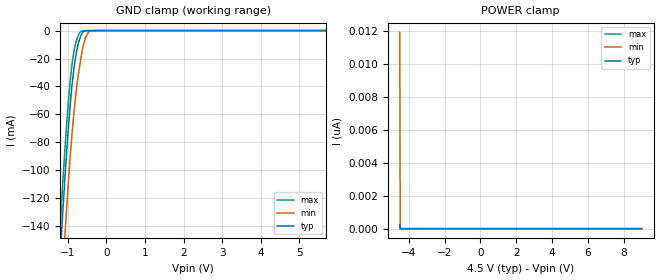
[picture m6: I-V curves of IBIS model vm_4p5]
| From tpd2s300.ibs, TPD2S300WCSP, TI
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|   VM_4p5 Model
[Model]   vm_4p5
Model_type   Input
Vinl = 1.35
Vinh = 3.15
|   typ   min   max
C_comp   15.123pF   11.1308pF   19.254pF
[Model spec]
|subparameter
Vinl   1.35   1.3497   1.3503
Vinh   3.15   3.1493   3.1507
| Where nom  PVT is Nominal Process, 4.5V, 27C
|   Fast PVT is Strong Process,  4.501V, -40C
|   Slow PVT is Weak Process,   4.499V, 125C
[Voltage Range]   4.5   4.499   4.501
[Temperature Range]   27   125   -40
[Power Clamp Reference]   4.5   4.499   4.501
[GND Clamp Reference]   0   0   0
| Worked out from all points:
|   GND clamp passes 1 mA (typ) near -0.60 V on its own axis
[GND Clamp]
|   Voltage   I(typ)   I(min)   I(max)
-4.5V     -1.887A    -2.023A    -1.826A
-1.26V    -189.6mA   -234.2mA   -167.6mA
-1.125V   -126.8mA   -169.1mA   -105.7mA
-1.058V   -97.56mA   -138.5mA   -77.21mA
-949.5mV  -56.44mA   -94.23mA   -38.92mA
-868.5mV  -33.11mA   -66.44mA   -19.36mA
-774mV    -15.04mA   -41.26mA   -6.877mA
-652.5mV  -3.023mA   -18.28mA   -456.3uA
-544.5mV  -166.6uA   -5.223mA   -12.33uA
-463.5mV  -10.66uA   -1.081mA   -920nA
-369mV    -33.47nA   -103.2uA   0A
9V        0A         0A         0A
[POWER Clamp]
|   Voltage   I(typ)   I(min)   I(max)
-4.5V     236.2pA    11.89nA    203.2pA
-4.473V   0A         0A         0A
-4.46V    0A         0A         0A
9V        0A         0A         0A
